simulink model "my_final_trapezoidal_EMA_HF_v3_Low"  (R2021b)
settings: Solver=FixedStepAuto  StartTime=0.0  StopTime=simulation.TiBr  FixedStep=simulation.DT  RelTol=1e-3  EnableMultiTasking=on
undefined symbols (not defined in the file or in its folder): BLDC, controller, DT, dynamics, inverter, simulation
libraries: fl_lib x22, nesl_utility x9, simulink x5, spsControlledVoltageSourceLib x3, spsCurrentMeasurementLib x3, spsSeriesRLCBranchLib x3, spsVoltageMeasurementLib x3, spsDCVoltageSourceLib x1, spsNeutralLib x1, spsUniversalBridgeLib x1, sdl_lib x1, spspowerguiLib x1

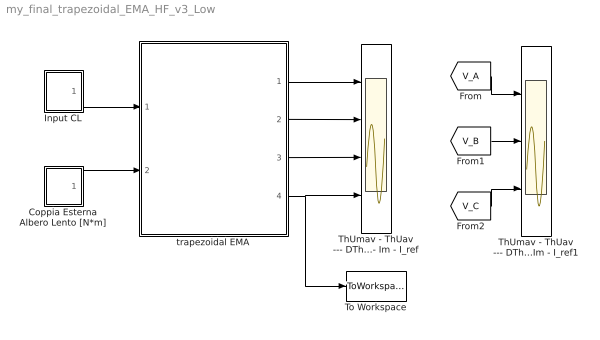
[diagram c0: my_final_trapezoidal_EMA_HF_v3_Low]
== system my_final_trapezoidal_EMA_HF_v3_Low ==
  Coppia Esterna Albero Lento [N*m] : Subsystem  mask(Coppia Esterna - Albero Lento - [N*m]){FRC0=0, FRC=0*0.25*BLDC.TMM, FRCt=0.1, FRR=0, FRR0=0, FRRt=4, FRA=0, FRSt=0, FRF=0}
      mask prompts: FRC0 "Valore iniziale TR (N*m):"; FRC "Coppia finale TRC (N*m):"; FRCt "Istante applicazione TRC (s):"; FRR "Pendenza rampa TR (N*m/s):"; FRR0 "Valore iniziale rampa TR (N*m):"; FRRt "Istante applicazione TRR (s):"; FRA "Ampiezza carico sinusoidale TRA (N*m):"; FRSt "Istante applicazione TRA (s):"; FRF "Frequenza FRA (Hz):"
      mask help: Forza Aerodinamica agente sulla superficie mobile mossa dal martinetto:
  Input CL : Subsystem  mask(Command Input:){IStep=off, IRamp=off, ISin=on, ICom=off, IChirp=off, INaTest=off, StepIni=0, StepFin=1%0.05%2%%0.01%0.05%0.1%0.5%1%, StepTime=0.01, RampTime=0, RampSlope=1e-3%5e-4%2%%5e-4%5e-2%5e-1%1, RampIC=0, SinAmp=0.1%%0.01%0.001%0.05, SinBias=0, SinFrq=1%%4*(2*pi)%10*(2*pi)%20*(2*pi)%50*(2*pi)%, ChirpAmp=0.005%0.025%0.005, ChirpIni=0, ChirpFrq=10, ChirpTg=0.5}
      mask prompts: IStep "Comando a Gradino (STEP)"; IRamp "Comando a Rampa (RAMP)"; ISin "Comando Sinusoidale (SIN)"; ICom "Time-History Comando (COM)"; IChirp "Comando Chirp (CHIRP)"; INaTest "Comando Test Na (TEST)"; StepIni "Ampiezza Iniziale [rad]:"; StepFin "Ampiezza Finale [rad]:"; StepTime "Istante Applic. Input [s]:"; RampTime "Istante Applic. Input [s]:"; RampSlope "Pendenza Rampa [rad/s]:"; RampIC "Output Iniziale Rampa [rad]:"; SinAmp "Semiampiezza Input [rad]:"; SinBias "Bias Input [rad]:"; SinFrq "Frequenza Input [rad/s]:"; ChirpAmp "Ampiezza Iniziale [rad]:"; ChirpIni "Frequenza Iniziale [Hz]:"; ChirpFrq "Frequenza di Target [Hz]:"; ChirpTg "Istante in cui raggiungo la Freq. di Target [s]:"
      mask help: Ricordati di settare correttamente i parametri relativi all'input selezionato prima di lanciare la simulazione!
  ThUmav - ThUav --- DThMm - DThM --- TMm - TM - TMm_lin - TM_lin --- I_refm - Im - I_ref : Scope  NumInputPorts=4
  ThUmav - ThUav --- DThMm - DThM --- TMm - TM - TMm_lin - TM_lin --- I_refm - Im - I_ref1 : Scope  NumInputPorts=3
  To Workspace : ToWorkspace  VariableName=iHF  SampleTime=-1
  trapezoidal EMA : Subsystem
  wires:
  Input CL/1(Out1) -> trapezoidal EMA/1(com)
  Coppia Esterna Albero Lento [N*m]/1(TR) -> trapezoidal EMA/2(load)
  trapezoidal EMA/1(theta_m) -> ThUmav - ThUav --- DThMm - DThM --- TMm - TM - TMm_lin - TM_lin --- I_refm - Im - I_ref/1
  trapezoidal EMA/2(Dtheta_m) -> ThUmav - ThUav --- DThMm - DThM --- TMm - TM - TMm_lin - TM_lin --- I_refm - Im - I_ref/2
  trapezoidal EMA/3(theta_u) -> ThUmav - ThUav --- DThMm - DThM --- TMm - TM - TMm_lin - TM_lin --- I_refm - Im - I_ref/3
  trapezoidal EMA/4(I_3eq) -> To Workspace/1, ThUmav - ThUav --- DThMm - DThM --- TMm - TM - TMm_lin - TM_lin --- I_refm - Im - I_ref/4
  [V_A] -> ThUmav - ThUav --- DThMm - DThM --- TMm - TM - TMm_lin - TM_lin --- I_refm - Im - I_ref1/1
  [V_B] -> ThUmav - ThUav --- DThMm - DThM --- TMm - TM - TMm_lin - TM_lin --- I_refm - Im - I_ref1/2
  [V_C] -> ThUmav - ThUav --- DThMm - DThM --- TMm - TM - TMm_lin - TM_lin --- I_refm - Im - I_ref1/3

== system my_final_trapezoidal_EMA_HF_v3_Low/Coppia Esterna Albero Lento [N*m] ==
  Clock : Clock
  Constant : Constant  Value=0
  FRC : Step  Time=FRCt  Before=FRC0  After=FRC  SampleTime=0
  FRR : simulink/Sources/Ramp  slope=FRR  start=FRRt  InitialOutput=FRR0
  FRS : Sin  Amplitude=FRA  Frequency=2*pi*FRF  Phase=-2*pi*FRF*FRSt  SampleTime=0
  Sum : Sum  Inputs=+++
  Switch : Switch  Threshold=FRSt
  TR : Outport
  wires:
  FRS/1 -> Switch/1
  Clock/1 -> Switch/2
  Constant/1 -> Switch/3
  Switch/1 -> Sum/3
  Sum/1 -> TR/1
  FRR/1 -> Sum/2
  FRC/1 -> Sum/1

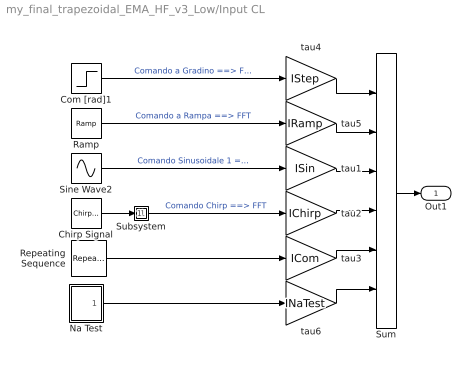
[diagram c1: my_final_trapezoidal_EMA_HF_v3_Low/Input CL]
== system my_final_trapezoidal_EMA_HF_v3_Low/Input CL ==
  Chirp Signal : simulink/Sources/Chirp Signal  f1=ChirpIni  T=ChirpTg  f2=ChirpFrq
  Com [rad]1 : Step  Time=StepTime  Before=StepIni  After=StepFin  SampleTime=0
  Na Test : Subsystem
  Ramp : simulink/Sources/Ramp  slope=RampSlope  start=RampTime  InitialOutput=RampIC
  Repeating Sequence : simulink/Sources/Repeating Sequence  rep_seq_t=simulation.timeCom  rep_seq_y=simulation.com
  Sine Wave2 : Sin  Amplitude=SinAmp  Bias=SinBias  Frequency=SinFrq  SampleTime=0
  Subsystem : Subsystem
  Sum : Sum  Inputs=++++++
  tau1 : Gain  Gain=ISin
  tau2 : Gain  Gain=IChirp
  tau3 : Gain  Gain=ICom
  tau4 : Gain  Gain=IStep
  tau5 : Gain  Gain=IRamp
  tau6 : Gain  Gain=INaTest
  Out1 : Outport
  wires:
  Com [rad]1/1 -> tau4/1  "Comando a Gradino ==> FFT"
  Sine Wave2/1 -> tau1/1  "Comando Sinusoidale 1 ==> r"
  Chirp Signal/1 -> Subsystem/1(In1)
  Subsystem/1(Out1) -> tau2/1  "Comando Chirp ==> FFT"
  Repeating Sequence/1 -> tau3/1
  tau4/1 -> Sum/1
  tau1/1 -> Sum/3
  tau2/1 -> Sum/4
  tau3/1 -> Sum/5
  Sum/1 -> Out1/1
  Ramp/1 -> tau5/1  "Comando a Rampa ==> FFT"
  tau5/1 -> Sum/2
  Na Test/1(Out) -> tau6/1
  tau6/1 -> Sum/6

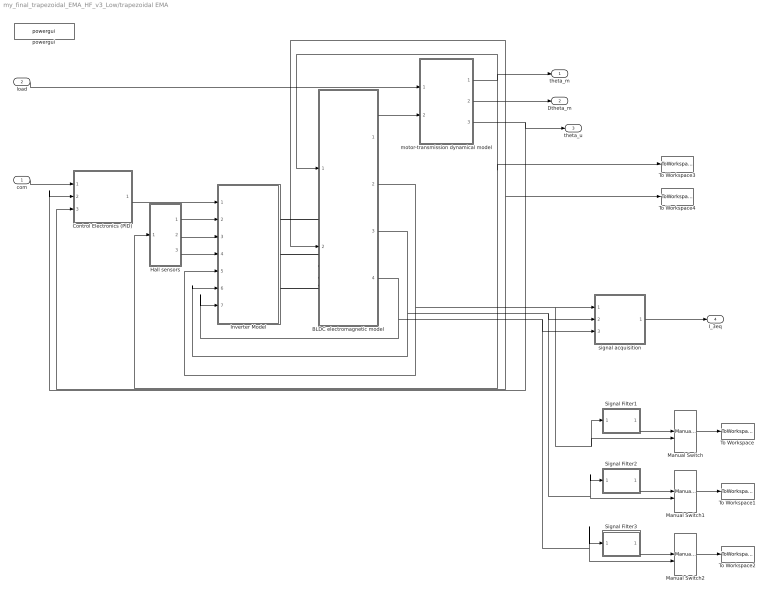
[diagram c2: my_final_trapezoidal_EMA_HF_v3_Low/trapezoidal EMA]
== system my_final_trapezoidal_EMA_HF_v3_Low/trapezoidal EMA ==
  com : Inport
  load : Inport  Port=2
  BLDC electromagnetic model : Subsystem
  Control Electronics (PID) : Subsystem
  Hall sensors : Subsystem
  Inverter Model : Subsystem
  Manual Switch : ManualSwitch
  Manual Switch1 : ManualSwitch
  Manual Switch2 : ManualSwitch
  Signal Filter1 : Subsystem  mask{tauF=simulation.tauFilter}
      mask prompts: tauF "Costante di tempo Filtro Passa-Basso [s]:"
  Signal Filter2 : Subsystem  mask{tauF=simulation.tauFilter}
      mask prompts: tauF "Costante di tempo Filtro Passa-Basso [s]:"
  Signal Filter3 : Subsystem  mask{tauF=simulation.tauFilter}
      mask prompts: tauF "Costante di tempo Filtro Passa-Basso [s]:"
  To Workspace : ToWorkspace  VariableName=IA  SampleTime=-1
  To Workspace1 : ToWorkspace  VariableName=IB  SampleTime=-1
  To Workspace2 : ToWorkspace  VariableName=IC  SampleTime=-1
  To Workspace3 : ToWorkspace  VariableName=thetaM  SampleTime=-1
  To Workspace4 : ToWorkspace  VariableName=Dtheta  SampleTime=-1
  motor-transmission dynamical model : Subsystem
  powergui : spspowerguiLib/powergui  Priority=1  SimulationMode=Continuous  SampleTime=DT  frequency=60  Iterations=50  frequencyindice=0  Pbase=100e6  ErrMax=1e-4  UnitsV=kV  UnitsW=MW  buscounter=0  FunctionMessages=on  echomessages=off  EnableUseOfTLC=off  CurrentSourceSwitches=off  DisableSnubberDevices=off  DisableRonSwitches=off  DisableVfSwitches=off  DisplayEquations=off  AutomaticDiscreteSolvers=off  SolverType=Tustin  Interpol=off  ExternalGateDelay=off  methode=off  Ts=10  x0status=blocks  SPID=off  SwTol=0  HookPort=off  NonlinearTolerance=1e-4  nMaxIteration=100  ContinueOnMaxIteration=off  RestoreLinks=no  ResistiveCurrentMeasurement=off  Frange=[0:2:500]  Ylog=off  Xlog=on  ShowGrid=off  save=off  variable=ZData  structure=0  ZoomFFT=off  StartTime=0.0  cycles=1  DisplayStyle=1  fundamental=60  FreqAxis=off  MaxFrequency=1000  frequencyindicesteady=1  RmsSteady=1  display=off
  signal acquisition : Subsystem
  theta_m : Outport
  Dtheta_m : Outport  Port=2
  theta_u : Outport  Port=3
  I_3eq : Outport  Port=4
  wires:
  Hall sensors/2(H2) -> Inverter Model/3(H2)
  com/1 -> Control Electronics (PID)/1(com [rad])
  motor-transmission dynamical model/3(theta_u) -> Control Electronics (PID)/2(theta_u [rad]), theta_u/1
  BLDC electromagnetic model/1(T_m) -> motor-transmission dynamical model/2(T_m)
  BLDC electromagnetic model/3(I_B) -> Inverter Model/6(I_B), signal acquisition/2(I_B), Signal Filter2/1(In1), Manual Switch1/2
  BLDC electromagnetic model/4(I_C) -> Inverter Model/7(I_C), signal acquisition/3(I_C), Signal Filter3/1(In1), Manual Switch2/2
  motor-transmission dynamical model/1(theta_m) -> Hall sensors/1(theta_m), To Workspace3/1, BLDC electromagnetic model/1(theta_m), theta_m/1
  load/1 -> motor-transmission dynamical model/1(load)
  signal acquisition/1(I_3eq) -> I_3eq/1
  Hall sensors/3(H3) -> Inverter Model/4(H3)
  Control Electronics (PID)/1(I_ref) -> Inverter Model/1(I_ref)
  motor-transmission dynamical model/2(Dtheta_m) -> To Workspace4/1, Control Electronics (PID)/3(Dtheta_m [rad]), BLDC electromagnetic model/2(Dtheta_m), Dtheta_m/1
  Hall sensors/1(H1) -> Inverter Model/2(H1)
  BLDC electromagnetic model/2(I_A) -> signal acquisition/1(I_A), Manual Switch/2, Signal Filter1/1(In1), Inverter Model/5(I_A)
  Signal Filter1/1(Out1) -> Manual Switch/1
  Manual Switch/1 -> To Workspace/1
  Signal Filter2/1(Out1) -> Manual Switch1/1
  Manual Switch2/1 -> To Workspace2/1
  Signal Filter3/1(Out1) -> Manual Switch2/1
  Manual Switch1/1 -> To Workspace1/1
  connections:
  BLDC electromagnetic model/LConn1 -- Inverter Model/RConn1
  BLDC electromagnetic model/LConn2 -- Inverter Model/RConn2
  BLDC electromagnetic model/LConn3 -- Inverter Model/RConn3

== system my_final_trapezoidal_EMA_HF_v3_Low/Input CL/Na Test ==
  IC : Constant  Value=0
  Sine Wave : Sin  Amplitude=0*0.005  Frequency=500*(2*pi)  SampleTime=0
  Step_1 : Step  Time=0.2  After=0*pi/3*dynamics.tau  SampleTime=0
  Step_2 : Step  Time=0.3  After=0*pi/3*dynamics.tau  SampleTime=0
  Sum : Sum  Inputs=|++
  Sum1 : Sum  Inputs=|++
  Sum2 : Sum  Inputs=|++
  Out : Outport
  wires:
  Sine Wave/1 -> Sum2/1
  Step_1/1 -> Sum/2
  Sum/1 -> Sum1/1
  Step_2/1 -> Sum1/2
  Sum1/1 -> Out/1
  Sum2/1 -> Sum/1
  IC/1 -> Sum2/2

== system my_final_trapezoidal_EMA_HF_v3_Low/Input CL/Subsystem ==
  In1 : Inport
  Clock : Clock
  Divide : Product  Inputs=*/
  Fcn : Fcn  Expr=exp(5*u/ChirpTg)
  Gain : Gain  Gain=ChirpAmp
  Manual Switch : ManualSwitch
  Saturation : Saturate  UpperLimit=inf  LowerLimit=1
  Out1 : Outport
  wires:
  Clock/1 -> Fcn/1
  In1/1 -> Divide/1, Manual Switch/1
  Divide/1 -> Manual Switch/2
  Saturation/1 -> Divide/2
  Fcn/1 -> Saturation/1
  Gain/1 -> Out1/1
  Manual Switch/1 -> Gain/1

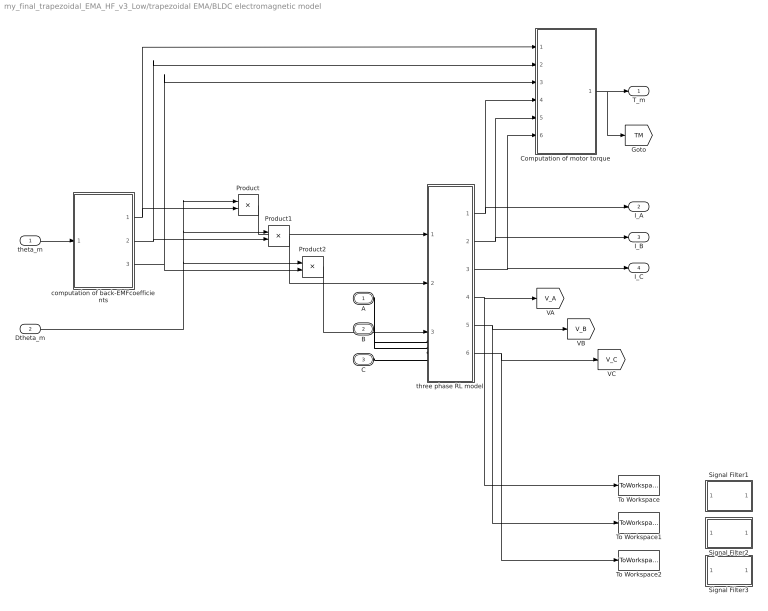
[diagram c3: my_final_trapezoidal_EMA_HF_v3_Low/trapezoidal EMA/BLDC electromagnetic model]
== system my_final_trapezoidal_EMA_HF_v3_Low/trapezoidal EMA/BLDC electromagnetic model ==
  theta_m : Inport
  Dtheta_m : Inport  Port=2
  Computation of motor torque : Subsystem
  Product : Product
  Product1 : Product
  Product2 : Product
  Signal Filter1 : Subsystem  mask{tauF=simulation.tauFilter}
      mask prompts: tauF "Costante di tempo Filtro Passa-Basso [s]:"
  Signal Filter2 : Subsystem  mask{tauF=simulation.tauFilter}
      mask prompts: tauF "Costante di tempo Filtro Passa-Basso [s]:"
  Signal Filter3 : Subsystem  mask{tauF=simulation.tauFilter}
      mask prompts: tauF "Costante di tempo Filtro Passa-Basso [s]:"
  To Workspace : ToWorkspace  VariableName=VA  SampleTime=-1
  To Workspace1 : ToWorkspace  VariableName=VB  SampleTime=-1
  To Workspace2 : ToWorkspace  VariableName=VC  SampleTime=-1
  computation of back-EMFcoefficients : Subsystem
  three phase RL model : Subsystem
  A : PMIOPort  Tag=PMCPort  Side=Left
  B : PMIOPort  Tag=PMCPort  Port=2  Side=Left
  C : PMIOPort  Tag=PMCPort  Port=3  Side=Left
  T_m : Outport
  I_A : Outport  Port=2
  I_B : Outport  Port=3
  I_C : Outport  Port=4
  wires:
  three phase RL model/1(I_A) -> Computation of motor torque/4(I_A), I_A/1
  three phase RL model/2(I_B) -> Computation of motor torque/5(I_B), I_B/1
  three phase RL model/3(I_C) -> Computation of motor torque/6(I_C), I_C/1
  theta_m/1 -> computation of back-EMFcoefficients/1(theta_m)
  Product/1 -> three phase RL model/1(E_A)
  Product1/1 -> three phase RL model/2(E_B)
  Product2/1 -> three phase RL model/3(E_C)
  Dtheta_m/1 -> Product/1, Product1/1, Product2/1
  computation of back-EMFcoefficients/1(k_A) -> Product/2, Computation of motor torque/1(k_A)
  computation of back-EMFcoefficients/2(k_B) -> Computation of motor torque/2(k_B), Product1/2
  computation of back-EMFcoefficients/3(k_C) -> Computation of motor torque/3(k_C), Product2/2
  Computation of motor torque/1(TM) -> [TM], T_m/1
  three phase RL model/5(V_B) -> To Workspace1/1, [V_B]
  three phase RL model/6(V_C) -> To Workspace2/1, [V_C]
  three phase RL model/4(V_A) -> To Workspace/1, [V_A]
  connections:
  A/RConn1 -- three phase RL model/LConn1
  B/RConn1 -- three phase RL model/LConn2
  three phase RL model/LConn3 -- C/RConn1

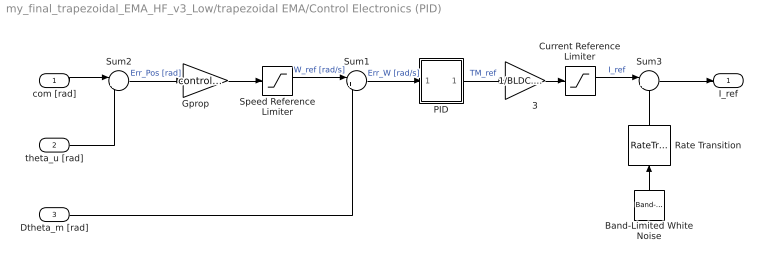
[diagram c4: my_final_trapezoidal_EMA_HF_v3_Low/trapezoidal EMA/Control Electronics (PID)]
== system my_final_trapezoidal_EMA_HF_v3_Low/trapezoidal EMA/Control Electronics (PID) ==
  com [rad] : Inport
  theta_u [rad] : Inport  Port=2
  Dtheta_m [rad] : Inport  Port=3
  "       3" : Gain  Gain=1/BLDC.Ke/2  SaturateOnIntegerOverflow=on
  Band-Limited White Noise : simulink/Sources/Band-Limited White Noise  Cov=controller.Knoise*[1e-6]  Ts=100*simulation.DT  seed=[0]
  Current Reference Limiter : Saturate  UpperLimit=controller.I_Max  LowerLimit=-controller.I_Max
  "Gprop       " : Gain  Gain=controller.Gprop  SaturateOnIntegerOverflow=on
  PID : Subsystem
  Rate Transition : RateTransition
  Speed Reference Limiter : Saturate  UpperLimit=controller.W_refMax  LowerLimit=-controller.W_refMax
  Sum1 : Sum  Inputs=|+-
  Sum2 : Sum  Inputs=|+-
  Sum3 : Sum  Inputs=|+-
  I_ref : Outport
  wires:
  Dtheta_m [rad]/1 -> Sum1/2
  Sum2/1 -> "Gprop       "/1  "Err_Pos [rad]"
  Speed Reference Limiter/1 -> Sum1/1  "W_ref [rad/s]"
  "Gprop       "/1 -> Speed Reference Limiter/1
  "       3"/1 -> Current Reference Limiter/1
  Current Reference Limiter/1 -> Sum3/1  "I_ref"
  Sum1/1 -> PID/1(Err_W)  "Err_W [rad/s]"
  PID/1(TMth) -> "       3"/1  "TM_ref"
  Sum3/1 -> I_ref/1
  Band-Limited White Noise/1 -> Rate Transition/1
  Rate Transition/1 -> Sum3/2
  com [rad]/1 -> Sum2/1
  theta_u [rad]/1 -> Sum2/2

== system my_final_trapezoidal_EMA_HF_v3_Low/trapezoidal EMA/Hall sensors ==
  theta_m : Inport
  Hall Sensor H1 : Lookup  InputValues=(pi/6)*[0 1 1 7 7 12]  Table=[1 1 0 0 1 1]
  Hall Sensor H2 : Lookup  InputValues=(pi/6)*[0 5 5 11 11 12]  Table=[1 1 0 0 1 1]
  Hall Sensor H3 : Lookup  InputValues=(pi/6)*[0 3 3 9 9 12]  Table=[0 0 1 1 0 0]
  computation of theta_e : Fcn  Expr=2*pi*(BLDC.P*u/2/pi - floor(BLDC.P*u/2/pi))
  H1 : Outport
  H2 : Outport  Port=2
  H3 : Outport  Port=3
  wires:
  theta_m/1 -> computation of theta_e/1
  computation of theta_e/1 -> Hall Sensor H2/1, Hall Sensor H1/1, Hall Sensor H3/1  "theta_e"
  Hall Sensor H1/1 -> H1/1
  Hall Sensor H2/1 -> H2/1
  Hall Sensor H3/1 -> H3/1

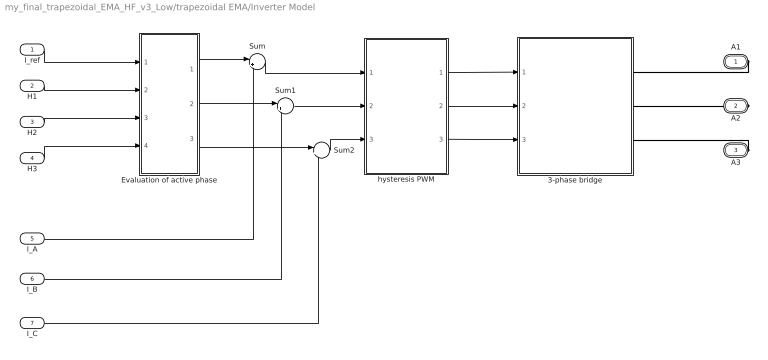
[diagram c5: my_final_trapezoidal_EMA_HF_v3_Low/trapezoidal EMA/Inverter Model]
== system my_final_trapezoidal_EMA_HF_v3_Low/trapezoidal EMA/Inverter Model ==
  I_ref : Inport
  H1 : Inport  Port=2
  H2 : Inport  Port=3
  H3 : Inport  Port=4
  I_A : Inport  Port=5
  I_B : Inport  Port=6
  I_C : Inport  Port=7
  3-phase bridge : Subsystem
  Evaluation of active phase : Subsystem
  Sum : Sum  Inputs=|+-
  Sum1 : Sum  Inputs=|+-
  Sum2 : Sum  Inputs=|+-
  hysteresis PWM : Subsystem
  A1 : PMIOPort  Tag=PMCPort  Side=Right
  A2 : PMIOPort  Tag=PMCPort  Port=2  Side=Right
  A3 : PMIOPort  Tag=PMCPort  Port=3  Side=Right
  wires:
  I_ref/1 -> Evaluation of active phase/1(I_ref)
  H1/1 -> Evaluation of active phase/2(H1)
  H2/1 -> Evaluation of active phase/3(H2)
  H3/1 -> Evaluation of active phase/4(H3)
  Evaluation of active phase/1(I_refA) -> Sum/1
  Evaluation of active phase/2(I_refB) -> Sum1/1
  Evaluation of active phase/3(I_refC) -> Sum2/1
  I_A/1 -> Sum/2
  I_B/1 -> Sum1/2
  I_C/1 -> Sum2/2
  Sum/1 -> hysteresis PWM/1(I_errA)
  Sum1/1 -> hysteresis PWM/2(I_errB)
  Sum2/1 -> hysteresis PWM/3(I_errC)
  hysteresis PWM/1(PWM_A) -> 3-phase bridge/1(PWM_A)
  hysteresis PWM/2(PWM_B) -> 3-phase bridge/2(PWM_B)
  hysteresis PWM/3(PWM_C) -> 3-phase bridge/3(PWM_C)
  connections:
  A1/RConn1 -- 3-phase bridge/RConn1
  A2/RConn1 -- 3-phase bridge/RConn2
  A3/RConn1 -- 3-phase bridge/RConn3

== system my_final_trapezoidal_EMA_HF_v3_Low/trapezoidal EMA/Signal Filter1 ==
  In1 : Inport
  Subsystem1 : Subsystem
  Out1 : Outport
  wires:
  In1/1 -> Subsystem1/1(In1)
  Subsystem1/1(Out1) -> Out1/1

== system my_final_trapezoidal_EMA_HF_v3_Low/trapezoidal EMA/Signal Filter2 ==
  In1 : Inport
  Subsystem1 : Subsystem
  Out1 : Outport
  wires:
  Subsystem1/1(Out1) -> Out1/1
  In1/1 -> Subsystem1/1(In1)

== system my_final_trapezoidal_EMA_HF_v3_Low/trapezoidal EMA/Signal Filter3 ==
  In1 : Inport
  Subsystem1 : Subsystem
  Out1 : Outport
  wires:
  In1/1 -> Subsystem1/1(In1)
  Subsystem1/1(Out1) -> Out1/1

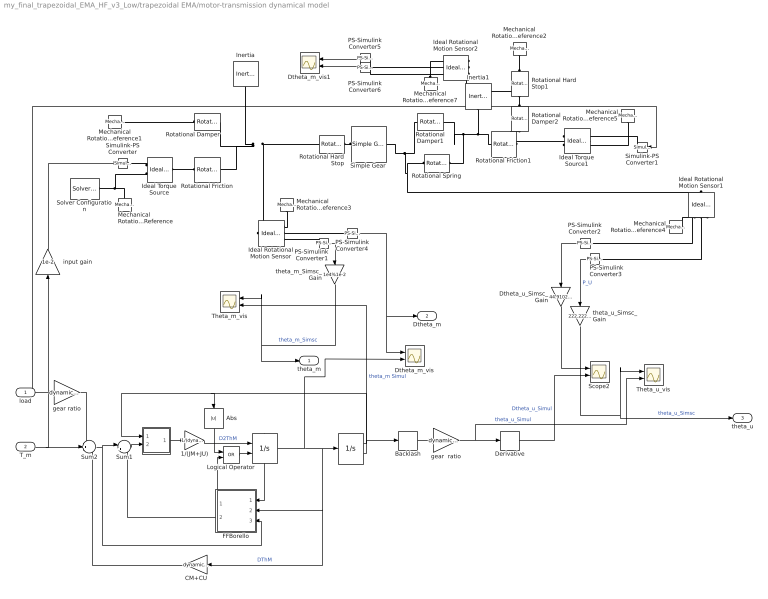
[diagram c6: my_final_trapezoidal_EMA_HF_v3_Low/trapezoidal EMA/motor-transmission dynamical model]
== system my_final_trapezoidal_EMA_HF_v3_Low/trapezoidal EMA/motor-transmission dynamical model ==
  load : Inport
  T_m : Inport  Port=2
  " " : Integrator  ExternalReset=rising  ShowStatePort=on
  "  " : Integrator  InitialCondition=simulation.initPos/dynamics.tau  LimitOutput=on  UpperSaturationLimit=dynamics.ThUmax/dynamics.tau  LowerSaturationLimit=dynamics.ThUmin/dynamics.tau  ShowSaturationPort=on
  "                       " : Subsystem
  1/(JM+JU) : Gain  Gain=1/(dynamics.JM+dynamics.JU)
  Abs : Abs
  Backlash : Backlash  BacklashWidth=dynamics.BLK/dynamics.tau
  CM+CU : Gain  Gain=dynamics.CM+dynamics.CU
  Derivative : Derivative
  Dtheta_m_vis : Scope  NumInputPorts=2
  Dtheta_m_vis1 : Scope  NumInputPorts=2
  Dtheta_u_Simsc_Gain : Gain  Gain=44.9102%1e-2
  FFBorello : Subsystem
  Ideal Rotational Motion Sensor : fl_lib/Mechanical/Mechanical Sensors/Ideal Rotational Motion Sensor  wrap_angle=simscape.enum.onoff.off  offset=0 rad
  Ideal Rotational Motion Sensor1 : fl_lib/Mechanical/Mechanical Sensors/Ideal Rotational Motion Sensor  wrap_angle=simscape.enum.onoff.off  offset=0 rad
  Ideal Rotational Motion Sensor2 : fl_lib/Mechanical/Mechanical Sensors/Ideal Rotational Motion Sensor  wrap_angle=simscape.enum.onoff.off  offset=0 rad
  Ideal Torque Source : fl_lib/Mechanical/Mechanical Sources/Ideal Torque Source
  Ideal Torque Source1 : fl_lib/Mechanical/Mechanical Sources/Ideal Torque Source
  Inertia : fl_lib/Mechanical/Rotational Elements/Inertia  inertia=dynamics.JM kg*m^2  num_ports=foundation.enum.numPorts2.one  w_specify=off  w_priority=High  w=0 rad/s  w_nominal_specify=off  w_nominal_unit=rad/s  w_nominal_value=1  t_specify=off  t_priority=None  t=0 N*m  t_nominal_specify=off  t_nominal_unit=N*m  t_nominal_value=1
  Inertia1 : fl_lib/Mechanical/Rotational Elements/Inertia  inertia=dynamics.JU kg*m^2  num_ports=foundation.enum.numPorts2.one  w_specify=off  w_priority=High  w=0 rad/s  w_nominal_specify=off  w_nominal_unit=rad/s  w_nominal_value=1  t_specify=off  t_priority=None  t=0 N*m  t_nominal_specify=off  t_nominal_unit=N*m  t_nominal_value=1
  Logical Operator : Logic  Operator=OR  AllPortsSameDT=off  OutDataTypeStr=boolean
  Mechanical Rotational Reference{,1..5,7} (7 alike) : fl_lib/Mechanical/Rotational Elements/Mechanical Rotational Reference
  PS-Simulink Converter{1..6} (6 alike) : nesl_utility/PS-Simulink Converter  PhysicalDomain=network_engine_domain  SubClassName=ps_output  LeftPortType=input  RightPortType=output  PseudoPeriodic=off  Frequencies=[]  Unit=inherit  AffineConversion=off
  Rotational Damper : fl_lib/Mechanical/Rotational Elements/Rotational Damper  D=dynamics.CM N*m/(rad/s)  w_specify=off  w_priority=None  w=0 rad/s  w_nominal_specify=off  w_nominal_unit=rad/s  w_nominal_value=1  t_specify=off  t_priority=None  t=0 N*m  t_nominal_specify=off  t_nominal_unit=N*m  t_nominal_value=1
  Rotational Damper1 : fl_lib/Mechanical/Rotational Elements/Rotational Damper  D=1 N*m/(rad/s)  w_specify=off  w_priority=None  w=0 rad/s  w_nominal_specify=off  w_nominal_unit=rad/s  w_nominal_value=1  t_specify=off  t_priority=None  t=0 N*m  t_nominal_specify=off  t_nominal_unit=N*m  t_nominal_value=1
  Rotational Damper2 : fl_lib/Mechanical/Rotational Elements/Rotational Damper  D=dynamics.CU N*m/(rad/s)  w_specify=off  w_priority=None  w=0 rad/s  w_nominal_specify=off  w_nominal_unit=rad/s  w_nominal_value=1  t_specify=off  t_priority=None  t=0 N*m  t_nominal_specify=off  t_nominal_unit=N*m  t_nominal_value=1
  Rotational Friction : fl_lib/Mechanical/Rotational Elements/Rotational Friction  brkwy_trq=0.06765 N*m  brkwy_vel=0.1 rad/s  Col_trq=0.03378 N*m  visc_coef=0 N*m/(rad/s)  w_specify=off  w_priority=None  w=0 rad/s  w_nominal_specify=off  w_nominal_unit=rad/s  w_nominal_value=1  t_specify=off  t_priority=None  t=0 N*m  t_nominal_specify=off  t_nominal_unit=N*m  t_nominal_value=1
  Rotational Friction1 : fl_lib/Mechanical/Rotational Elements/Rotational Friction  brkwy_trq=0.06765 N*m  brkwy_vel=0.1 rad/s  Col_trq=0.03378 N*m  visc_coef=0 N*m/(rad/s)  w_specify=off  w_priority=None  w=0 rad/s  w_nominal_specify=off  w_nominal_unit=rad/s  w_nominal_value=1  t_specify=off  t_priority=None  t=0 N*m  t_nominal_specify=off  t_nominal_unit=N*m  t_nominal_value=1
  Rotational Hard Stop : fl_lib/Mechanical/Rotational Elements/Rotational Hard Stop  upper_bnd=dynamics.BLK/dynamics.tau rad  lower_bnd=-dynamics.BLK/dynamics.tau rad  stiff_up=1e6 N*m/rad  stiff_low=1e6 N*m/rad  D_up=0.01 N*m/(rad/s)  D_low=0.01 N*m/(rad/s)  model=simscape.enum.hardstop.smooth  transition=0.001 rad  w_specify=off  w_priority=None  w=0 rad/s  w_nominal_specify=off  w_nominal_unit=rad/s  w_nominal_value=1  t_specify=off  t_priority=None  t=0 N*m  t_nominal_specify=off  t_nominal_unit=N*m  t_nominal_value=1  phi_specify=off  phi_priority=High  phi=0 rad  phi_nominal_specify=off  phi_nominal_unit=rad  phi_nominal_value=1
  Rotational Hard Stop1 : fl_lib/Mechanical/Rotational Elements/Rotational Hard Stop  upper_bnd=dynamics.ThUmax rad  lower_bnd=dynamics.ThUmin rad  stiff_up=1e6 N*m/rad  stiff_low=1e6 N*m/rad  D_up=0.01 N*m/(rad/s)  D_low=0.01 N*m/(rad/s)  model=simscape.enum.hardstop.smooth  transition=0.001 rad  w_specify=off  w_priority=None  w=0 rad/s  w_nominal_specify=off  w_nominal_unit=rad/s  w_nominal_value=1  t_specify=off  t_priority=None  t=0 N*m  t_nominal_specify=off  t_nominal_unit=N*m  t_nominal_value=1  phi_specify=off  phi_priority=High  phi=0 rad  phi_nominal_specify=off  phi_nominal_unit=rad  phi_nominal_value=1
  Rotational Spring : fl_lib/Mechanical/Rotational Elements/Rotational Spring  spr_rate=1 N*m/rad  w_specify=off  w_priority=None  w=0 rad/s  w_nominal_specify=off  w_nominal_unit=rad/s  w_nominal_value=1  t_specify=off  t_priority=None  t=0 N*m  t_nominal_specify=off  t_nominal_unit=N*m  t_nominal_value=1  phi_specify=off  phi_priority=High  phi=0 rad  phi_nominal_specify=off  phi_nominal_unit=rad  phi_nominal_value=1
  Scope2 : Scope  NumInputPorts=2
  Simple Gear : sdl_lib/Gears/Simple Gear  ratio=dynamics.tau  rotation_direction=sdl.enum.shaftOutputDirection.same  friction_model=sdl.enum.gear_efficiencies_load.off  T_noload=0.1 N*m  T_nom=5 N*m  efficiency_nom=0.8  efficiency=0.8  temperature_TLU=[280, 300, 320] K  load_TLU=[1, 5, 10] N*m  efficiency_TLU=[.95, .9, .85]  efficiency_TLU2=[.85, .8, .75; .95, .9, .85; .85, .8, .7]  w_thr=0.01 rad/s  pwr_thr=0.001 W  backlash_model=sdl.enum.backlashModel.Off  backlash_distance=1e-3 mm  x0=0 mm  r_base=0.1 m  hardstop_model=simscape.enum.hardstop.smooth  transition=1e-4 mm  backlash_stiffness=1e7 N/m  backlash_damping=1e6 N/(m/s)  e=0  v_tol=0.001 m/s  mu_visc=[0, 0] N*m/(rad/s)  enable_faults=simscape.enum.onoff.off  efficiency_fault=0.05  external_fault=simscape.enum.onoff.off  temporal_fault=simscape.enum.onoff.off  fault_time=5 s  fault_angles=pi / 12 rad  report_fault=simscape.enum.assert.action.none  thermal_mass=50 J/K  temperature_specify=off  temperature_priority=High  temperature=300 K  temperature_nominal_specify=off  temperature_nominal_unit=K  temperature_nominal_value=1  x_backlash_specify=off  x_backlash_priority=None  x_backlash=0 mm  x_backlash_nominal_specify=off  x_backlash_nominal_unit=mm  x_backlash_nominal_value=1  f_hardstop_specify=off  f_hardstop_priority=None  f_hardstop=0 N  f_hardstop_nominal_specify=off  f_hardstop_nominal_unit=N  f_hardstop_nominal_value=1  v_backlash_specify=off  v_backlash_priority=None  v_backlash=0 m/s  v_backlash_nominal_specify=off  v_backlash_nominal_unit=m/s  v_backlash_nominal_value=1
  Simulink-PS Converter : nesl_utility/Simulink-PS Converter  PhysicalDomain=network_engine_domain  SubClassName=ps_input  LeftPortType=input  RightPortType=output  PseudoPeriodic=off  Frequencies=[]  NoiseDistribution=none  NoiseParameters=[]  Unit=1  AffineConversion=off  FilteringAndDerivatives=provide  SimscapeFilterOrder=1  InputFilterTimeConstant=0.001  UdotUserProvided=0
  Simulink-PS Converter1 : nesl_utility/Simulink-PS Converter  PhysicalDomain=network_engine_domain  SubClassName=ps_input  LeftPortType=input  RightPortType=output  PseudoPeriodic=off  Frequencies=[]  NoiseDistribution=none  NoiseParameters=[]  Unit=1  AffineConversion=off  FilteringAndDerivatives=provide  SimscapeFilterOrder=1  InputFilterTimeConstant=0.001  UdotUserProvided=0
  Solver Configuration : nesl_utility/Solver Configuration  PhysicalDomain=network_engine_domain  SubClassName=solver  LeftPortType=input  RightPortType=generic  Tones=[]  Harmonics=[]  SimulateNoise=off  Profile=off  UseLocalSampling=off  EnableSwitchedLinearOptims=on  FrequencyDomain=off  UseCCode=off  RelTol=0.001  AbsTol=1e-06  MinStep=1e-09  ToWorkspace=off  RevertToSquareIcSolve=off  NumHomotopyIterations=100  PhasorMode=off  PhasorModeNumHarmonics=1  DoDC=off  ResidualTolerance=1e-09  UseLocalSolver=off  LocalSolverChoice=NE_BACKWARD_EULER_ADVANCER  LocalSolverSampleTime=0.001  DoFixedCost=off  MaxNonlinIter=3  MaxModeIter=2  ComputeImpulses=off  ImpulseIterations=2  LinearAlgebra=auto  EquationFormulation=NE_TIME_EF  DelaysMemoryBudget=1024  AutomaticFiltering=on  FilteringTimeConstant=0.001  PartitionStorageMethod=AS_NEEDED  PartitionMemoryBudget=1024  PartitionMethod=ROBUST
  Sum1 : Sum  Inputs=|+-
  Sum2 : Sum  Inputs=-+-
  Theta_m_vis : Scope  NumInputPorts=2
  Theta_u_vis : Scope  NumInputPorts=2
  gear  ratio : Gain  Gain=dynamics.tau
  gear ratio : Gain  Gain=dynamics.tau
  input gain : Gain  Gain=1e-2
  theta_m_Simsc_Gain : Gain  Gain=1e4%1e-2
  theta_u_Simsc_Gain : Gain  Gain=222.222%66.666667
  theta_m : Outport
  Dtheta_m : Outport  Port=2
  theta_u : Outport  Port=3
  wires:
  1/(JM+JU)/1 -> " "/1  "D2ThM"
  CM+CU/1 -> Sum2/3
  Sum2/1 -> Sum1/1, FFBorello/3(Act Torque)
  Logical Operator/1 -> " "/2
  FFBorello/1(Reset_DXJ) -> Logical Operator/2
  Abs/1 -> Logical Operator/1
  "  "/2 -> Abs/1, "                       "/1(Sat Port)
  " "/State -> FFBorello/1(DThU SP)
  FFBorello/2(TF) -> Sum1/2
  Sum1/1 -> "                       "/2(Act ThC)
  "                       "/1(Act) -> 1/(JM+JU)/1
  "  "/1 -> Backlash/1, Theta_m_vis/2  "theta_m Simul"
  T_m/1 -> Sum2/2, input gain/1
  " "/1 -> Dtheta_m_vis/2, "  "/1, CM+CU/1, FFBorello/2(DThU)  "DThM"
  gear ratio/1 -> Sum2/1
  Backlash/1 -> gear  ratio/1
  load/1 -> gear ratio/1, Simulink-PS Converter1/1
  input gain/1 -> Simulink-PS Converter/1
  gear  ratio/1 -> Theta_u_vis/2, Derivative/1  "theta_u_Simul"
  Derivative/1 -> Scope2/2  "Dtheta_u_Simul"
  PS-Simulink Converter3/1 -> theta_u_Simsc_Gain/1  "P_U"
  PS-Simulink Converter2/1 -> Dtheta_u_Simsc_Gain/1
  theta_u_Simsc_Gain/1 -> theta_u/1, Theta_u_vis/1  "theta_u_Simsc"
  Dtheta_u_Simsc_Gain/1 -> Scope2/1
  PS-Simulink Converter4/1 -> Dtheta_m_vis/1, Dtheta_m/1
  PS-Simulink Converter1/1 -> theta_m_Simsc_Gain/1
  theta_m_Simsc_Gain/1 -> theta_m/1, Theta_m_vis/1  "theta_m_Simsc"
  PS-Simulink Converter6/1 -> Dtheta_m_vis1/2
  PS-Simulink Converter5/1 -> Dtheta_m_vis1/1
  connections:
  Rotational Friction1/RConn1 -- Ideal Torque Source1/LConn1 -- Rotational Damper2/RConn1
  Inertia1/LConn1 -- Rotational Friction1/LConn1 -- Rotational Spring/RConn1 -- Rotational Damper1/RConn1
  Ideal Rotational Motion Sensor1/LConn1 -- Simple Gear/RConn1 -- Rotational Damper1/LConn1 -- Rotational Spring/LConn1
  Solver Configuration/RConn1 -- Ideal Torque Source/RConn2 -- Mechanical Rotational Reference/LConn1
  Ideal Torque Source/RConn1 -- Simulink-PS Converter/RConn1
  Mechanical Rotational Reference3/LConn1 -- Ideal Rotational Motion Sensor/RConn1
  Rotational Hard Stop/RConn1 -- Simple Gear/LConn1
  PS-Simulink Converter2/LConn1 -- Ideal Rotational Motion Sensor1/RConn2
  PS-Simulink Converter1/LConn1 -- Ideal Rotational Motion Sensor/RConn3
  Rotational Friction/LConn1 -- Ideal Torque Source/LConn1
  PS-Simulink Converter4/LConn1 -- Ideal Rotational Motion Sensor/RConn2
  Mechanical Rotational Reference4/LConn1 -- Ideal Rotational Motion Sensor1/RConn1
  Mechanical Rotational Reference5/LConn1 -- Ideal Torque Source1/RConn2
  Simulink-PS Converter1/RConn1 -- Ideal Torque Source1/RConn1
  PS-Simulink Converter3/LConn1 -- Ideal Rotational Motion Sensor1/RConn3
  Ideal Rotational Motion Sensor/LConn1 -- Rotational Hard Stop/LConn1 -- Rotational Damper/RConn1 -- Rotational Friction/RConn1 -- Inertia/LConn1
  PS-Simulink Converter6/LConn1 -- Ideal Rotational Motion Sensor2/RConn2
  Mechanical Rotational Reference7/LConn1 -- Ideal Rotational Motion Sensor2/RConn1
  PS-Simulink Converter5/LConn1 -- Ideal Rotational Motion Sensor2/RConn3
  Rotational Damper/LConn1 -- Mechanical Rotational Reference1/LConn1
  Rotational Hard Stop1/LConn1 -- Mechanical Rotational Reference2/LConn1
  Rotational Hard Stop1/RConn1 -- Ideal Rotational Motion Sensor2/LConn1 -- Rotational Damper2/LConn1

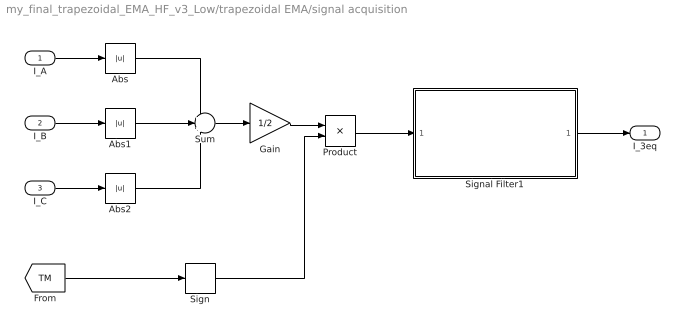
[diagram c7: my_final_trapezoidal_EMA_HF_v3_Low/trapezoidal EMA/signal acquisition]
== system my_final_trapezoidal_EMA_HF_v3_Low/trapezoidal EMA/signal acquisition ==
  I_A : Inport
  I_B : Inport  Port=2
  I_C : Inport  Port=3
  Abs : Abs
  Abs1 : Abs
  Abs2 : Abs
  Gain : Gain  Gain=1/2
  Product : Product  RndMeth=Zero
  Sign : Signum
  Signal Filter1 : Subsystem  mask{tauF=simulation.tauFilter}
      mask prompts: tauF "Costante di tempo Filtro Passa-Basso [s]:"
  Sum : Sum  Inputs=+++
  I_3eq : Outport
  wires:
  Abs/1 -> Sum/1
  Abs1/1 -> Sum/2
  Abs2/1 -> Sum/3
  Sum/1 -> Gain/1
  Gain/1 -> Product/1
  Sign/1 -> Product/2
  I_A/1 -> Abs/1
  I_B/1 -> Abs1/1
  I_C/1 -> Abs2/1
  Product/1 -> Signal Filter1/1(In1)
  [TM] -> Sign/1
  Signal Filter1/1(Out1) -> I_3eq/1

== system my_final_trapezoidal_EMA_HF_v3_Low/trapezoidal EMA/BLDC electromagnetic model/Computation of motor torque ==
  note: Inserire il modello termico del BLDC e relazionare ke_a con la temperatura
  note: e_in = FCEM_i normalizzata = ei / DThM
  k_A : Inport
  k_B : Inport  Port=2
  k_C : Inport  Port=3
  I_A : Inport  Port=4
  I_B : Inport  Port=5
  I_C : Inport  Port=6
  Add2 : Sum  Inputs=+++
  Product : Product
  Product1 : Product
  Product2 : Product
  TMM : Saturate  UpperLimit=BLDC.TMM  LowerLimit=-BLDC.TMM
  TM : Outport
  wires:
  TMM/1 -> TM/1
  Add2/1 -> TMM/1
  I_A/1 -> Product/2
  k_A/1 -> Product/1
  Product/1 -> Add2/1
  Product1/1 -> Add2/2
  I_B/1 -> Product1/2
  k_B/1 -> Product1/1
  Product2/1 -> Add2/3
  k_C/1 -> Product2/1
  I_C/1 -> Product2/2

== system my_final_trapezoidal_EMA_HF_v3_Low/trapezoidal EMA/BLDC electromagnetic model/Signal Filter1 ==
  In1 : Inport
  Subsystem1 : Subsystem
  Out1 : Outport
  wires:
  In1/1 -> Subsystem1/1(In1)
  Subsystem1/1(Out1) -> Out1/1

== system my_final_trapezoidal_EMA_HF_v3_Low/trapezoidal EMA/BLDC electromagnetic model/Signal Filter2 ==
  In1 : Inport
  Subsystem1 : Subsystem
  Out1 : Outport
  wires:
  Subsystem1/1(Out1) -> Out1/1
  In1/1 -> Subsystem1/1(In1)

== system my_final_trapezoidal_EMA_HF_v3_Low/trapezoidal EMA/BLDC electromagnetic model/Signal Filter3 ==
  In1 : Inport
  Subsystem1 : Subsystem
  Out1 : Outport
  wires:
  In1/1 -> Subsystem1/1(In1)
  Subsystem1/1(Out1) -> Out1/1

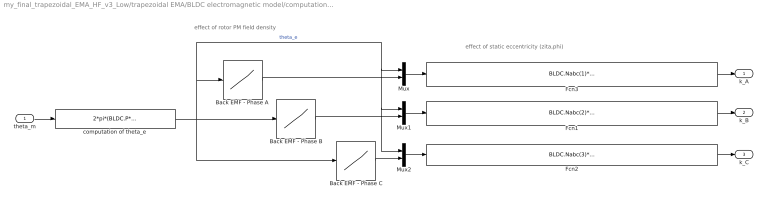
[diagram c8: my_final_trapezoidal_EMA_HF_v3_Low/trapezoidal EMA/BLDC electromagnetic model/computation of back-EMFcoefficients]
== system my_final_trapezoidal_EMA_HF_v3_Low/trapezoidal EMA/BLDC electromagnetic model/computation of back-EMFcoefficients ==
  note: effect of rotor PM field density
  note: effect of static eccentricity (zita,phi)
  theta_m : Inport
  Back EMF - Phase A : Lookup  InputValues=(pi/6)*[0 1 1 3 5 5 7 7 9 11 11 12]  Table=[0 0 1 1 1 0 0 -1 -1 -1 0 0]
  Back EMF - Phase B : Lookup  InputValues=(pi/6)*[0 1 3 3 5 5 7 9 9 11 11 12]  Table=[-1 -1 -1 0 0 1 1 1 0 0 -1 -1]
  Back EMF - Phase C : Lookup  InputValues=(pi/6)*[0 1 1 3 3 5 7 7 9 9 11 12]  Table=[1 1 0 0 -1 -1 -1 0 0 1 1 1]
  Fcn1 : Fcn  Expr=BLDC.Nabc(2)*BLDC.Ke*u(2)*(1+(BLDC.P>1)*BLDC.zeta*cos(u(1)-BLDC.phi+2*pi/3))
  Fcn2 : Fcn  Expr=BLDC.Nabc(3)*BLDC.Ke*u(2)*(1+(BLDC.P>1)*BLDC.zeta*cos(u(1)-BLDC.phi+4*pi/3))
  Fcn3 : Fcn  Expr=BLDC.Nabc(1)*BLDC.Ke*u(2)*(1+(BLDC.P>1)*BLDC.zeta*cos(u(1)-BLDC.phi))
  Mux : Mux  Inputs=2
  Mux1 : Mux  Inputs=2
  Mux2 : Mux  Inputs=2
  computation of theta_e : Fcn  Expr=2*pi*(BLDC.P*u/2/pi - floor(BLDC.P*u/2/pi))
  k_A : Outport
  k_B : Outport  Port=2
  k_C : Outport  Port=3
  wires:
  Mux/1 -> Fcn3/1
  Fcn3/1 -> k_A/1
  Mux1/1 -> Fcn1/1
  Mux2/1 -> Fcn2/1
  Fcn1/1 -> k_B/1
  Fcn2/1 -> k_C/1
  Back EMF - Phase A/1 -> Mux/2
  Back EMF - Phase B/1 -> Mux1/2
  Back EMF - Phase C/1 -> Mux2/2
  theta_m/1 -> computation of theta_e/1
  computation of theta_e/1 -> Back EMF - Phase C/1, Mux/1, Mux1/1, Mux2/1, Back EMF - Phase A/1, Back EMF - Phase B/1  "theta_e"

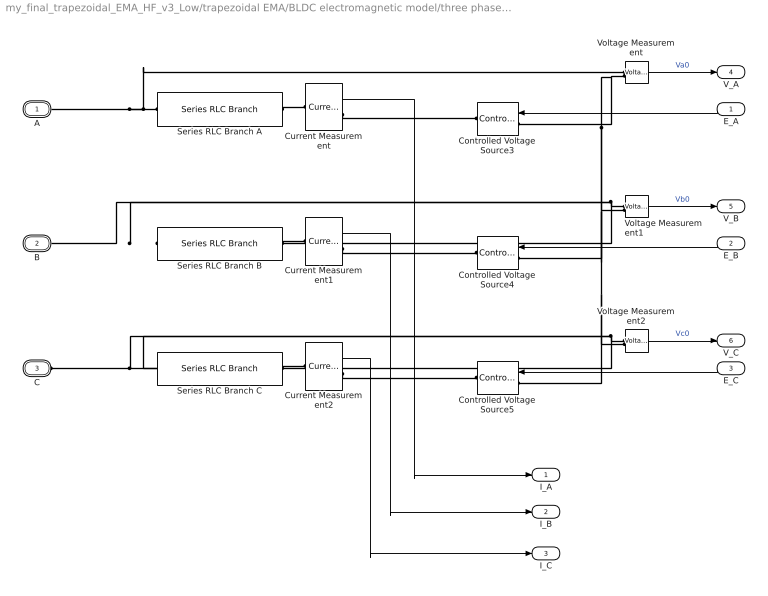
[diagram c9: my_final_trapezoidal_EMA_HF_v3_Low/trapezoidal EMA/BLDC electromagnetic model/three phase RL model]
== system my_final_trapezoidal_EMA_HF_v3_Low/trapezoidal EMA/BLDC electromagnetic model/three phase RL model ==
  E_A : Inport
  E_B : Inport  Port=2
  E_C : Inport  Port=3
  Controlled Voltage Source3 : spsControlledVoltageSourceLib/Controlled Voltage Source  Initialize=off  Source_Type=DC  Amplitude=0  Phase=0  Frequency=0  Measurements=None
  Controlled Voltage Source4 : spsControlledVoltageSourceLib/Controlled Voltage Source  Initialize=off  Source_Type=DC  Amplitude=0  Phase=0  Frequency=0  Measurements=None
  Controlled Voltage Source5 : spsControlledVoltageSourceLib/Controlled Voltage Source  Initialize=off  Source_Type=DC  Amplitude=0  Phase=0  Frequency=0  Measurements=None
  Current Measurement : spsCurrentMeasurementLib/Current Measurement  Tag=PoWeRsYsTeMmEaSuReMeNt  PhasorSimulation=off  OutputType=Magnitude  PSBequivalent=0
  Current Measurement1 : spsCurrentMeasurementLib/Current Measurement  Tag=PoWeRsYsTeMmEaSuReMeNt  PhasorSimulation=off  OutputType=Magnitude  PSBequivalent=0
  Current Measurement2 : spsCurrentMeasurementLib/Current Measurement  Tag=PoWeRsYsTeMmEaSuReMeNt  PhasorSimulation=off  OutputType=Magnitude  PSBequivalent=0
  Series RLC Branch A : spsSeriesRLCBranchLib/Series RLC Branch  LConnTagsString=__new0  RConnTagsString=__new0  BranchType=RL  Resistance=0.5*BLDC.Rs*BLDC.Nabc(1)  Inductance=0.5*BLDC.Ls*BLDC.Nabc(1)^2  SetiL0=off  InitialCurrent=0  Capacitance=1e-6  Setx0=off  InitialVoltage=0  Measurements=None
  Series RLC Branch B : spsSeriesRLCBranchLib/Series RLC Branch  LConnTagsString=__new0  RConnTagsString=__new0  BranchType=RL  Resistance=0.5*BLDC.Rs*BLDC.Nabc(2)  Inductance=0.5*BLDC.Ls*BLDC.Nabc(2)^2  SetiL0=off  InitialCurrent=0  Capacitance=1e-6  Setx0=off  InitialVoltage=0  Measurements=None
  Series RLC Branch C : spsSeriesRLCBranchLib/Series RLC Branch  LConnTagsString=__new0  RConnTagsString=__new0  BranchType=RL  Resistance=0.5*BLDC.Rs*BLDC.Nabc(3)  Inductance=0.5*BLDC.Ls*BLDC.Nabc(3)^2  SetiL0=off  InitialCurrent=0  Capacitance=1e-6  Setx0=off  InitialVoltage=0  Measurements=None
  Voltage Measurement : spsVoltageMeasurementLib/Voltage Measurement  PhasorSimulation=off  OutputType=Complex  PSBequivalent=0
  Voltage Measurement1 : spsVoltageMeasurementLib/Voltage Measurement  PhasorSimulation=off  OutputType=Complex  PSBequivalent=0
  Voltage Measurement2 : spsVoltageMeasurementLib/Voltage Measurement  PhasorSimulation=off  OutputType=Complex  PSBequivalent=0
  A : PMIOPort  Tag=PMCPort  Side=Left
  B : PMIOPort  Tag=PMCPort  Port=2  Side=Left
  C : PMIOPort  Tag=PMCPort  Port=3  Side=Left
  I_A : Outport
  I_B : Outport  Port=2
  I_C : Outport  Port=3
  V_A : Outport  Port=4
  V_B : Outport  Port=5
  V_C : Outport  Port=6
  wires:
  Voltage Measurement/1 -> V_A/1  "Va0"
  Voltage Measurement2/1 -> V_C/1  "Vc0"
  Voltage Measurement1/1 -> V_B/1  "Vb0"
  Current Measurement/1 -> I_A/1
  Current Measurement1/1 -> I_B/1
  E_A/1 -> Controlled Voltage Source3/1
  Current Measurement2/1 -> I_C/1
  E_C/1 -> Controlled Voltage Source5/1
  E_B/1 -> Controlled Voltage Source4/1
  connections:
  Voltage Measurement1/LConn1 -- B/RConn1 -- Series RLC Branch B/LConn1
  Series RLC Branch A/LConn1 -- A/RConn1 -- Voltage Measurement/LConn1
  Series RLC Branch B/RConn1 -- Current Measurement1/LConn1
  Series RLC Branch A/RConn1 -- Current Measurement/LConn1
  Current Measurement/RConn1 -- Controlled Voltage Source3/RConn1
  Current Measurement2/RConn1 -- Controlled Voltage Source5/RConn1
  Current Measurement1/RConn1 -- Controlled Voltage Source4/RConn1
  Series RLC Branch C/RConn1 -- Current Measurement2/LConn1
  Voltage Measurement/LConn2 -- Controlled Voltage Source5/LConn1 -- Voltage Measurement2/LConn2 -- Controlled Voltage Source4/LConn1 -- Voltage Measurement1/LConn2 -- Controlled Voltage Source3/LConn1
  Voltage Measurement2/LConn1 -- C/RConn1 -- Series RLC Branch C/LConn1

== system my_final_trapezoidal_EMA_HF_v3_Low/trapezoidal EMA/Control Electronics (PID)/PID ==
  Err_W : Inport
  Filter : Integrator  DisableCoverage=on
  GAD : Gain  Gain=controller.PID.GAD
  GAI : Gain  Gain=controller.PID.GAI
  GAP : Gain  Gain=controller.PID.GAP
  Integrator : Integrator  DisableCoverage=on  LimitOutput=on  UpperSaturationLimit=controller.PID.ErIM  LowerSaturationLimit=-controller.PID.ErIM
  N : Gain  Gain=1000
  Sum : Sum  Inputs=+++
  Sum1 : Sum  Inputs=|+-
  TMth : Outport
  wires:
  GAP/1 -> Sum/1
  GAI/1 -> Integrator/1
  GAD/1 -> Sum1/1
  Sum1/1 -> N/1
  N/1 -> Filter/1, Sum/3
  Filter/1 -> Sum1/2
  Integrator/1 -> Sum/2
  Err_W/1 -> GAP/1, GAI/1, GAD/1
  Sum/1 -> TMth/1

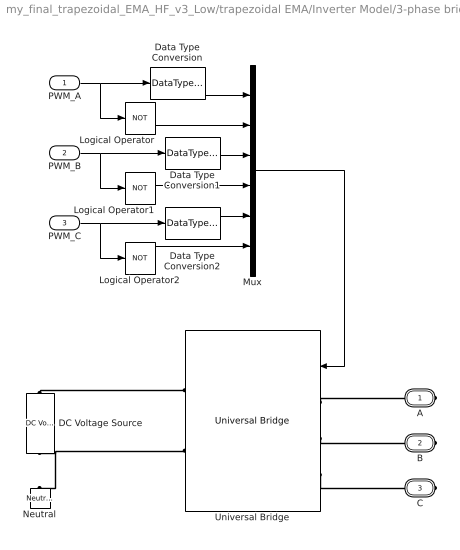
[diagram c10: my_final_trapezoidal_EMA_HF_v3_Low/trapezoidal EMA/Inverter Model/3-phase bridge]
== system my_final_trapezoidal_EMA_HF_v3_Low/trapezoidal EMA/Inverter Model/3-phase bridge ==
  PWM_A : Inport
  PWM_B : Inport  Port=2
  PWM_C : Inport  Port=3
  DC Voltage Source : spsDCVoltageSourceLib/DC Voltage Source  Amplitude=inverter.Hbridge.Vdc  Measurements=None
  Data Type Conversion : DataTypeConversion  OutDataTypeStr=boolean
  Data Type Conversion1 : DataTypeConversion  OutDataTypeStr=boolean
  Data Type Conversion2 : DataTypeConversion  OutDataTypeStr=boolean
  Logical Operator : Logic  Operator=NOT  AllPortsSameDT=off
  Logical Operator1 : Logic  Operator=NOT  AllPortsSameDT=off
  Logical Operator2 : Logic  Operator=NOT  AllPortsSameDT=off
  Mux : Mux  Inputs=6
  Neutral : spsNeutralLib/Neutral  LConnTagsString=a  NodeNumber=0
  Universal Bridge : spsUniversalBridgeLib/Universal Bridge  Arms=3  SnubberResistance=inverter.Hbridge.RSnubber  SnubberCapacitance=inverter.Hbridge.CSnubber  Device=MOSFET / Diodes  Ron=inverter.Hbridge.Ron  Lon=0  ForwardVoltages="[  0  0  ]"  ForwardVoltage=0  GTOparameters=[ 10e-6 , 20e-6 ]  IGBTparameters=[ 1e-6 , 2e-6 ]  Measurements=None  Measurements_2=None  converterType=Rectifier
  A : PMIOPort  Tag=PMCPort  Side=Right
  B : PMIOPort  Tag=PMCPort  Port=2  Side=Right
  C : PMIOPort  Tag=PMCPort  Port=3  Side=Right
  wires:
  PWM_A/1 -> Logical Operator/1, Data Type Conversion/1
  Logical Operator/1 -> Mux/2
  PWM_B/1 -> Logical Operator1/1, Data Type Conversion1/1
  Logical Operator1/1 -> Mux/4
  PWM_C/1 -> Logical Operator2/1, Data Type Conversion2/1
  Logical Operator2/1 -> Mux/6
  Mux/1 -> Universal Bridge/1
  Data Type Conversion/1 -> Mux/1
  Data Type Conversion1/1 -> Mux/3
  Data Type Conversion2/1 -> Mux/5
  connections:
  DC Voltage Source/RConn1 -- Universal Bridge/RConn1
  Universal Bridge/RConn2 -- Neutral/LConn1 -- DC Voltage Source/LConn1
  Universal Bridge/LConn1 -- A/RConn1
  Universal Bridge/LConn2 -- B/RConn1
  Universal Bridge/LConn3 -- C/RConn1

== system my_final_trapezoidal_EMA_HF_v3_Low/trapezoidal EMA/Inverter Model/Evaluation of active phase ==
  I_ref : Inport
  H1 : Inport  Port=2
  H2 : Inport  Port=3
  H3 : Inport  Port=4
  H1 - H3 : Sum  Inputs=-+
  H2 - H1 : Sum  Inputs=-+
  H3 - H2 : Sum  Inputs=-+
  Product : Product  RndMeth=Zero
  Product1 : Product  RndMeth=Zero
  Product2 : Product  RndMeth=Zero
  I_refA : Outport
  I_refB : Outport  Port=2
  I_refC : Outport  Port=3
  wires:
  I_ref/1 -> Product2/1, Product1/1, Product/1
  Product/1 -> I_refA/1
  Product1/1 -> I_refB/1
  Product2/1 -> I_refC/1
  H1 - H3/1 -> Product2/2  "C"
  H2/1 -> H3 - H2/1, H2 - H1/2
  H1/1 -> H1 - H3/2, H2 - H1/1
  H2 - H1/1 -> Product/2  "A"
  H3 - H2/1 -> Product1/2  "B"
  H3/1 -> H1 - H3/1, H3 - H2/2  "C"

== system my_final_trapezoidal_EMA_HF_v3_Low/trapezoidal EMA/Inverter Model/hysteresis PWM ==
  I_errA : Inport
  I_errB : Inport  Port=2
  I_errC : Inport  Port=3
  Relay : Relay  OnSwitchValue=inverter.PWM.hb  OffSwitchValue=-inverter.PWM.hb
  Relay1 : Relay  OnSwitchValue=inverter.PWM.hb  OffSwitchValue=-inverter.PWM.hb
  Relay2 : Relay  OnSwitchValue=inverter.PWM.hb  OffSwitchValue=-inverter.PWM.hb
  PWM_A : Outport
  PWM_B : Outport  Port=2
  PWM_C : Outport  Port=3
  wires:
  I_errA/1 -> Relay/1
  I_errB/1 -> Relay1/1
  I_errC/1 -> Relay2/1
  Relay1/1 -> PWM_B/1
  Relay2/1 -> PWM_C/1
  Relay/1 -> PWM_A/1

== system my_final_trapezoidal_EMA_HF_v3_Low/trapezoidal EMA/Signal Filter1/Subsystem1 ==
  In1 : Inport
  Transfer Fcn1 : TransferFcn  Denominator=[tauF 1]
  Transfer Fcn3 : TransferFcn  Numerator=1  Denominator=[tauF 1]
  Transfer Fcn4 : TransferFcn  Numerator=1  Denominator=[tauF 1]
  Out1 : Outport
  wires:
  Transfer Fcn1/1 -> Transfer Fcn3/1
  Transfer Fcn3/1 -> Transfer Fcn4/1
  In1/1 -> Transfer Fcn1/1
  Transfer Fcn4/1 -> Out1/1

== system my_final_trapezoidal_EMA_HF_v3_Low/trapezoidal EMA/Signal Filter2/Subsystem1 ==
  In1 : Inport
  Transfer Fcn1 : TransferFcn  Denominator=[tauF 1]
  Transfer Fcn3 : TransferFcn  Numerator=1  Denominator=[tauF 1]
  Transfer Fcn4 : TransferFcn  Numerator=1  Denominator=[tauF 1]
  Out1 : Outport
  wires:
  Transfer Fcn4/1 -> Out1/1
  In1/1 -> Transfer Fcn1/1
  Transfer Fcn3/1 -> Transfer Fcn4/1
  Transfer Fcn1/1 -> Transfer Fcn3/1

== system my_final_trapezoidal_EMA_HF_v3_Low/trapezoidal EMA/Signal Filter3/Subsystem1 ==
  In1 : Inport
  Transfer Fcn1 : TransferFcn  Denominator=[tauF 1]
  Transfer Fcn3 : TransferFcn  Numerator=1  Denominator=[tauF 1]
  Transfer Fcn4 : TransferFcn  Numerator=1  Denominator=[tauF 1]
  Out1 : Outport
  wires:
  Transfer Fcn1/1 -> Transfer Fcn3/1
  Transfer Fcn3/1 -> Transfer Fcn4/1
  In1/1 -> Transfer Fcn1/1
  Transfer Fcn4/1 -> Out1/1

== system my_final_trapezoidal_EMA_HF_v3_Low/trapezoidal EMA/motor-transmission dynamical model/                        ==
  Sat Port : Inport
  Act ThC : Inport  Port=2
  "    " : Constant  Value=0
  Product : Product  RndMeth=Zero
  Sign : Signum
  Switch : Switch  Threshold=0.5
  Act : Outport
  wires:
  Act ThC/1 -> Switch/3, Sign/1
  Product/1 -> Switch/2
  Sign/1 -> Product/2
  "    "/1 -> Switch/1
  Switch/1 -> Act/1
  Sat Port/1 -> Product/1

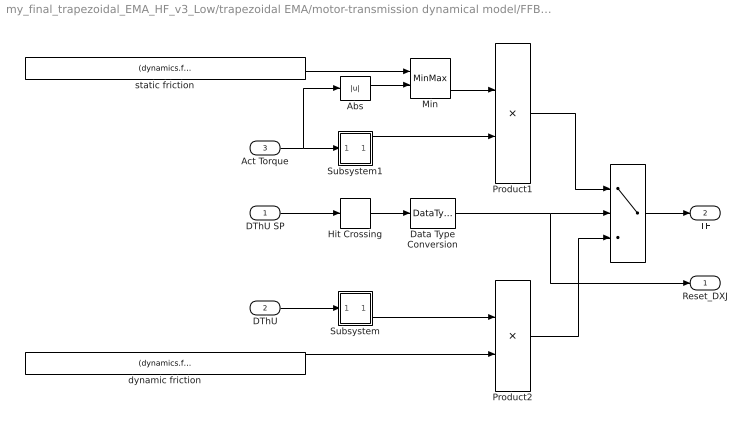
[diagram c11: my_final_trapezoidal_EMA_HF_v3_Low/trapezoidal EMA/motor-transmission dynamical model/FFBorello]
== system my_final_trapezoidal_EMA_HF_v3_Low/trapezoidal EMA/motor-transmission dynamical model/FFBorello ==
  DThU SP : Inport
  DThU : Inport  Port=2
  Act Torque : Inport  Port=3
  "   " : Switch  Threshold=0.5
  Abs : Abs
  Data Type Conversion : DataTypeConversion  OutDataTypeStr=double
  Hit Crossing : HitCross
  Min : MinMax  Inputs=2  InputSameDT=on  SaturateOnIntegerOverflow=on
  Product1 : Product  InputSameDT=on  RndMeth=Zero  SaturateOnIntegerOverflow=on
  Product2 : Product  InputSameDT=on  RndMeth=Zero  SaturateOnIntegerOverflow=on
  Subsystem : Subsystem
  Subsystem1 : Subsystem
  dynamic friction : Constant  Value=(dynamics.friction.FDTm+dynamics.friction.FDTu)*BLDC.TMM
  static friction : Constant  Value=(dynamics.friction.FSTm+dynamics.friction.FSTu)*BLDC.TMM
  Reset_DXJ : Outport
  TF : Outport  Port=2
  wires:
  Product2/1 -> "   "/3
  DThU/1 -> Subsystem/1(In1)
  "   "/1 -> TF/1
  Product1/1 -> "   "/1
  Min/1 -> Product1/1
  Act Torque/1 -> Subsystem1/1(In1), Abs/1
  Abs/1 -> Min/2
  Hit Crossing/1 -> Data Type Conversion/1
  Subsystem/1(Out1) -> Product2/1
  Subsystem1/1(Out1) -> Product1/2
  Data Type Conversion/1 -> "   "/2, Reset_DXJ/1
  DThU SP/1 -> Hit Crossing/1
  static friction/1 -> Min/1
  dynamic friction/1 -> Product2/2

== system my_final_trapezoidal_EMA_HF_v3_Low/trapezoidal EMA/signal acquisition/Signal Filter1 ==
  In1 : Inport
  Subsystem1 : Subsystem
  Out1 : Outport
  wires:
  In1/1 -> Subsystem1/1(In1)
  Subsystem1/1(Out1) -> Out1/1

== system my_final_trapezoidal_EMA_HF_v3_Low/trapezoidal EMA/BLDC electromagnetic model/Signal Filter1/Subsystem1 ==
  In1 : Inport
  Transfer Fcn1 : TransferFcn  Denominator=[tauF 1]
  Transfer Fcn3 : TransferFcn  Numerator=1  Denominator=[tauF 1]
  Transfer Fcn4 : TransferFcn  Numerator=1  Denominator=[tauF 1]
  Out1 : Outport
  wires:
  Transfer Fcn1/1 -> Transfer Fcn3/1
  Transfer Fcn3/1 -> Transfer Fcn4/1
  In1/1 -> Transfer Fcn1/1
  Transfer Fcn4/1 -> Out1/1

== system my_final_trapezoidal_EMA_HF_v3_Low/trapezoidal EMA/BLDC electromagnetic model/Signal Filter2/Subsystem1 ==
  In1 : Inport
  Transfer Fcn1 : TransferFcn  Denominator=[tauF 1]
  Transfer Fcn3 : TransferFcn  Numerator=1  Denominator=[tauF 1]
  Transfer Fcn4 : TransferFcn  Numerator=1  Denominator=[tauF 1]
  Out1 : Outport
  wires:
  Transfer Fcn4/1 -> Out1/1
  In1/1 -> Transfer Fcn1/1
  Transfer Fcn3/1 -> Transfer Fcn4/1
  Transfer Fcn1/1 -> Transfer Fcn3/1

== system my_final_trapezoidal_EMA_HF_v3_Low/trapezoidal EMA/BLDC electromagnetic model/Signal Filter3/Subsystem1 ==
  In1 : Inport
  Transfer Fcn1 : TransferFcn  Denominator=[tauF 1]
  Transfer Fcn3 : TransferFcn  Numerator=1  Denominator=[tauF 1]
  Transfer Fcn4 : TransferFcn  Numerator=1  Denominator=[tauF 1]
  Out1 : Outport
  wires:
  Transfer Fcn1/1 -> Transfer Fcn3/1
  Transfer Fcn3/1 -> Transfer Fcn4/1
  In1/1 -> Transfer Fcn1/1
  Transfer Fcn4/1 -> Out1/1

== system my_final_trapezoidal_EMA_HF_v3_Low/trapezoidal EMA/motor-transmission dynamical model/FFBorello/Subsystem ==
  In1 : Inport
  "   2" : Switch
  FSJ [N]3 : Constant
  FSJ [N]4 : Constant  Value=-1
  Out1 : Outport
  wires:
  FSJ [N]3/1 -> "   2"/1
  FSJ [N]4/1 -> "   2"/3
  In1/1 -> "   2"/2
  "   2"/1 -> Out1/1

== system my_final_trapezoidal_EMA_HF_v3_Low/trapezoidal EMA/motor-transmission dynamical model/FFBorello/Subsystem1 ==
  In1 : Inport
  "   2" : Switch
  FSJ [N]3 : Constant
  FSJ [N]4 : Constant  Value=-1
  Out1 : Outport
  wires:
  FSJ [N]3/1 -> "   2"/1
  FSJ [N]4/1 -> "   2"/3
  In1/1 -> "   2"/2
  "   2"/1 -> Out1/1

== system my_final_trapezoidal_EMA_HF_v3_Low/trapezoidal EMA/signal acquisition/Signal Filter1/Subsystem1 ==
  In1 : Inport
  Transfer Fcn1 : TransferFcn  Denominator=[tauF 1]
  Transfer Fcn3 : TransferFcn  Numerator=1  Denominator=[tauF 1]
  Transfer Fcn4 : TransferFcn  Numerator=1  Denominator=[tauF 1]
  Out1 : Outport
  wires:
  Transfer Fcn1/1 -> Transfer Fcn3/1
  Transfer Fcn3/1 -> Transfer Fcn4/1
  In1/1 -> Transfer Fcn1/1
  Transfer Fcn4/1 -> Out1/1
